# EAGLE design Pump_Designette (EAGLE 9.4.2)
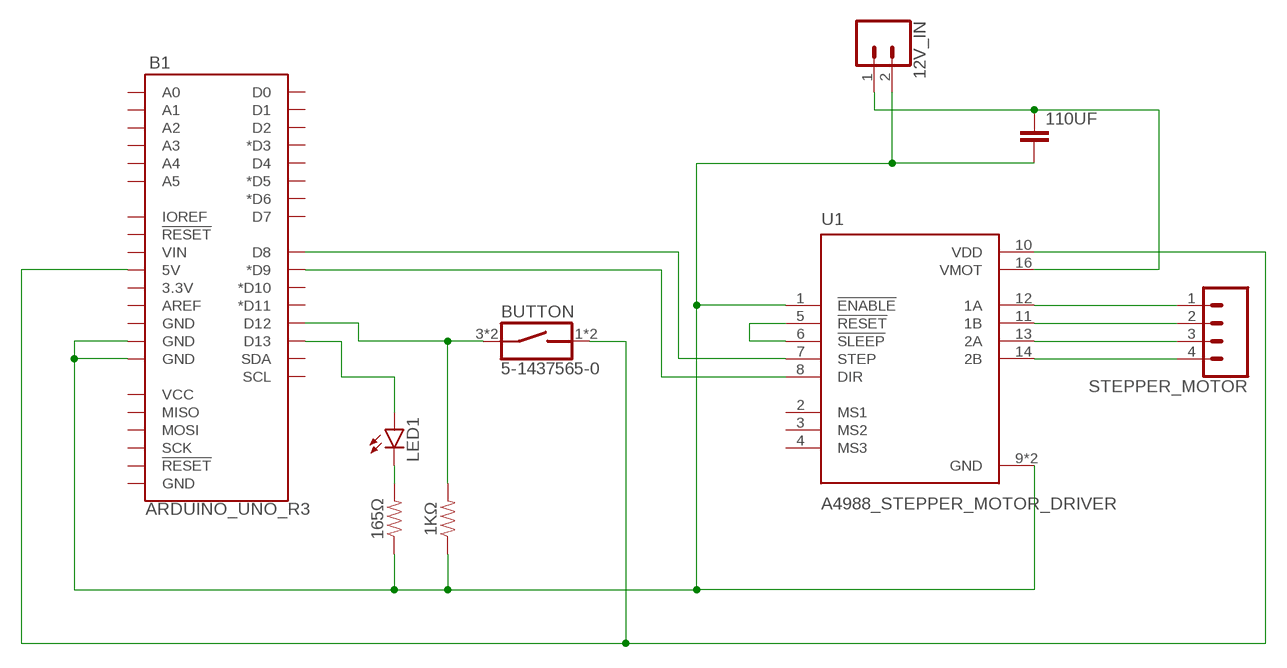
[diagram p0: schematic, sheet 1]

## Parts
1KΩ  1k  1KOHM-HORIZ-1/4W-1%  [AXIAL-0.3]
12V_IN  CONN_02  [1X02]
110UF  C2,5-3  [C2.5-3]
165Ω  1k  1KOHM-HORIZ-1/4W-1%  [AXIAL-0.3]
B1  ARDUINO_UNO_R3  [ARDUINO_R3]
BUTTON  5-1437565-0  [SW_5-1437565-0]
LED1  LED5MM  [LED5MM]
STEPPER_MOTOR  CONN_04  [1X04]
U1  A4988_STEPPER_MOTOR_DRIVER  A4988_STEPPER_MOTOR_DRIVER_CARRIER  [MODULE_A4988_STEPPER_MOTOR_DRIVER_CARRIER]

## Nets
N$1: 1KΩ.P$1 12V_IN.2 110UF.2 165Ω.P$1 B1.GND@2(GND) B1.GND@3(GND) U1.1(!ENABLE) U1.9(GND) U1.15(GND)
N$2: U1.5(!RESET) U1.6(!SLEEP)
N$3: B1.D9(*D9) U1.8(DIR)
N$4: B1.D8 U1.7(STEP)
N$5: STEPPER_MOTOR.1 U1.12(1A)
N$6: STEPPER_MOTOR.2 U1.11(1B)
N$7: STEPPER_MOTOR.3 U1.13(2A)
N$8: STEPPER_MOTOR.4 U1.14(2B)
N$9: 12V_IN.1 110UF.1 U1.16(VMOT)
N$10: B1.5V BUTTON.1 BUTTON.2 U1.10(VDD)
N$11: B1.D13 LED1.A
N$12: 1KΩ.P$2 B1.D12 BUTTON.3 BUTTON.4
N$13: 165Ω.P$2 LED1.K(C)
Unconnected: B1.3.3V B1.A0 B1.A1 B1.A2 B1.A3 B1.A4 B1.A5 B1.AREF B1.D0 B1.D1 B1.D2 B1.D3(*D3) B1.D4 B1.D5(*D5) B1.D6(*D6) B1.D7 B1.D10(*D10) B1.D11(*D11) B1.GND@1(GND) B1.GND@4(GND) B1.IOREF B1.MISO B1.MOSI B1.RESET@1(!RESET!) B1.RESET@2(!RESET!) B1.SCK B1.SCL B1.SDA B1.VCC B1.VIN U1.2(MS1) U1.3(MS2) U1.4(MS3)

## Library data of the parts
1KΩ 165Ω = SparkFun-Resistors:1KOHM: 1kΩ resistor; PROD_ID: RES-12182
12V_IN = SparkFun-Connectors:CONN_02: Multi connection point. Often used as Generic Header-pin footprint for 0.1 inch spaced/style header connections
110UF = capacitor-wima:C: CAPACITOR
B1 = SparkFun-Boards:ARDUINO_UNO_R3: Arduino R3 Footprint with SPI header Arduino Uno R3 Compatible Footprint. Matches PCB size of the original board. SparkFun Products: SAMD21 Dev Breakout RedBoard R3 Stackable Headers
BUTTON = 5-1437565-0:5-1437565-0: Switch Tactile OFF (ON) Round Button Gull Wing 0.05A 12VDC 1.57N SMD T/R; AVAILABILITY: Unavailable; COMMENT: 5-1437565-0; DESCRIPTION: Switch Push Button N.O. SPST Round Button 0.05A 12VDC 1VA Alternate Contact Gull Wing SMD T/R; MF: TE Connectivity; MP: FSM6JSMATR; PACKAGE: None; PRICE: None; TE_PURCHASE_URL: https://www.te.com/usa-en/product-5-1437565-0.html?te_bu=Cor&te_type=disp&te_campaign=seda_glo_cor-seda-global-disp-prtnr-fy19-seda-model-bom-cta_sma-317_1&elqCampaignId=32493
LED1 = led:LED: LED
STEPPER_MOTOR = SparkFun-Connectors:CONN_04: Multi connection point. Often used as Generic Header-pin footprint for 0.1 inch spaced/style header connections On any of the 0.1 inch spaced packages, you can populate with these: Break Away Headers - Straight (PRT-00116) Break Away Male Headers - Right Angle (PRT-00553) Female Headers (PRT-00115)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; PROD_ID: CONN-09696
U1 = A4988_STEPPER_MOTOR_DRIVER_CARRIER:A4988_STEPPER_MOTOR_DRIVER_CARRIER: Stepper motor controler; IC: A4988; 1A; Uin mot: 8÷35V; AVAILABILITY: Unavailable; DESCRIPTION: Stepper Motor Driver; MF: Pololu; MP: A4988 STEPPER MOTOR DRIVER CARRIER; PACKAGE: None; PRICE: None

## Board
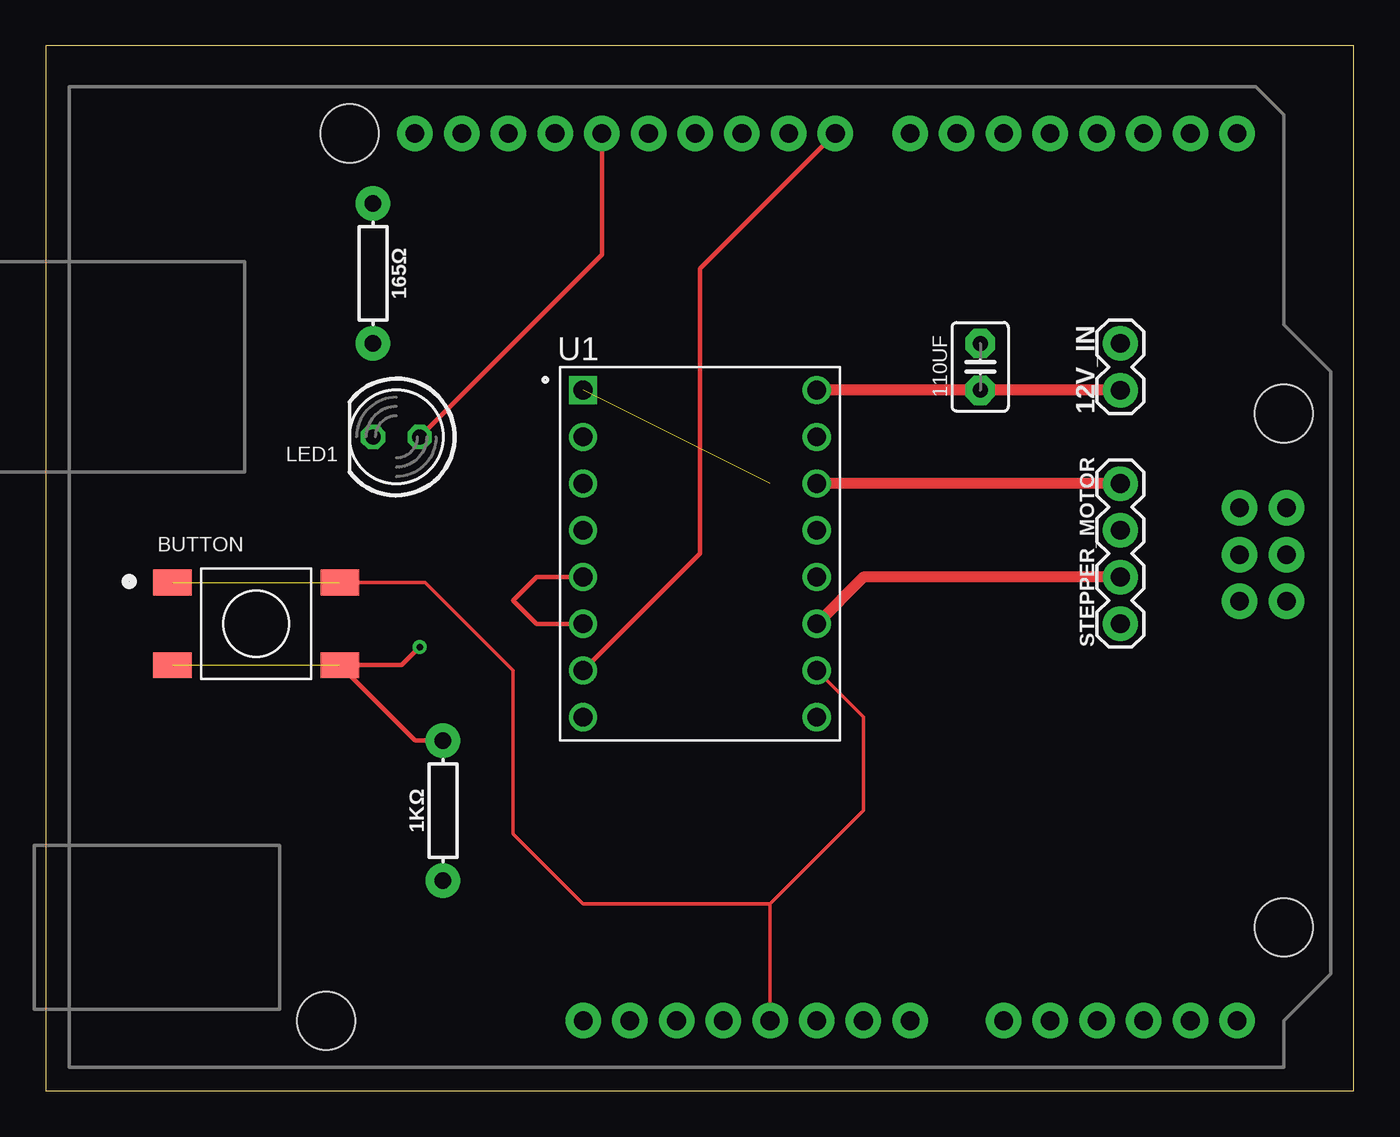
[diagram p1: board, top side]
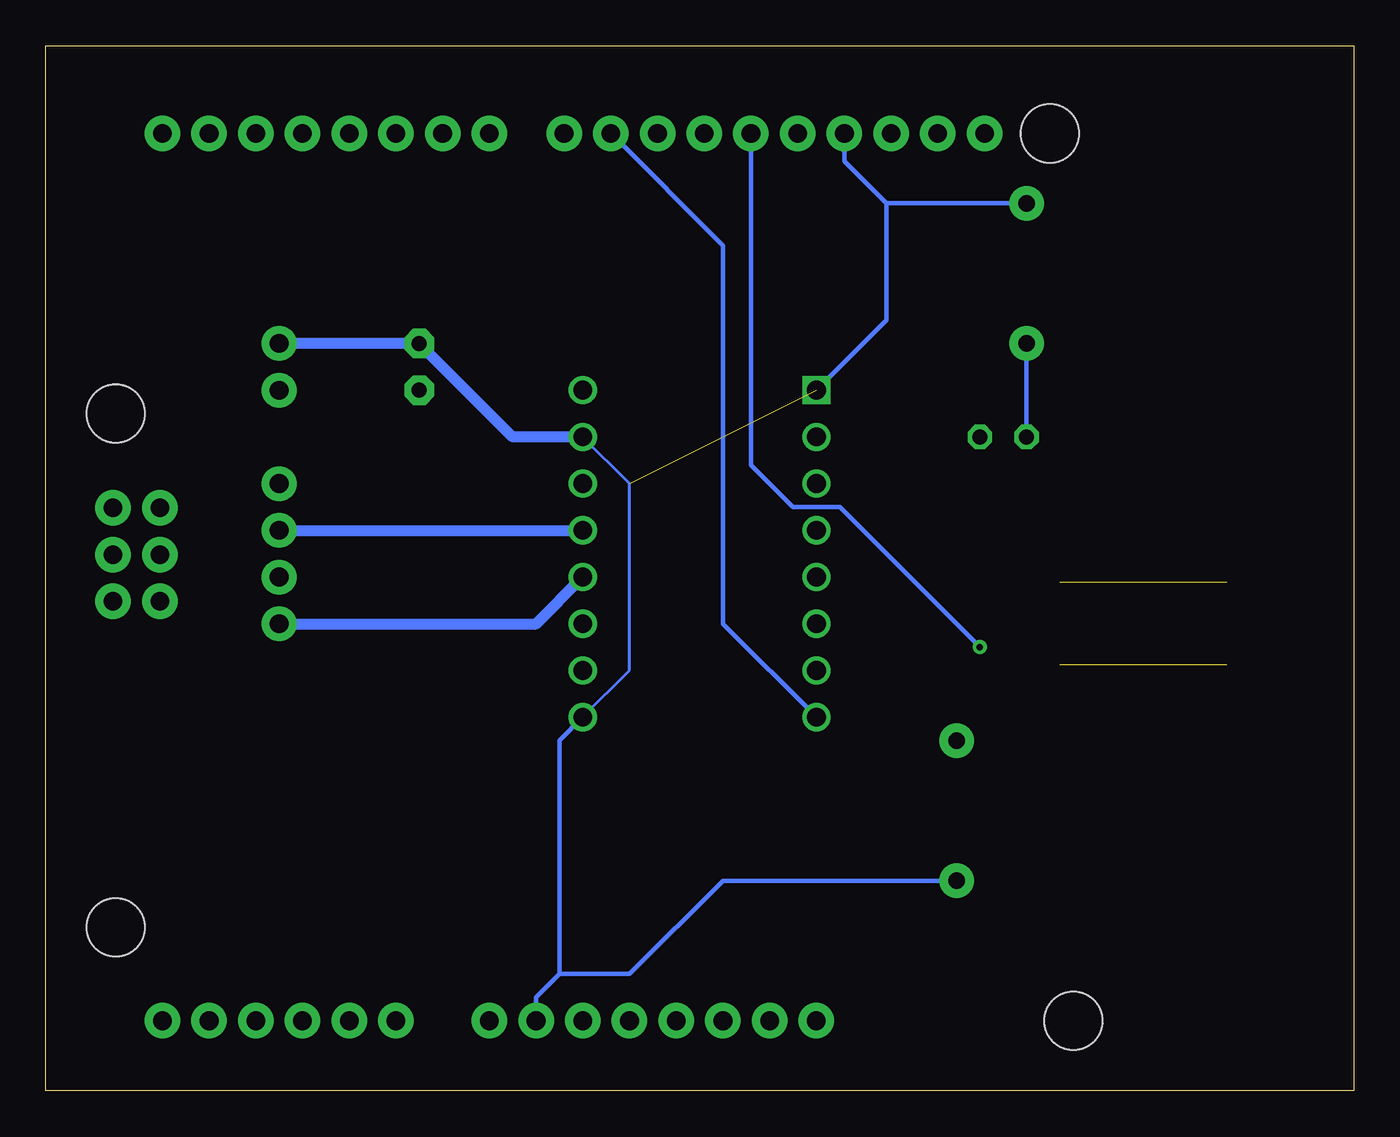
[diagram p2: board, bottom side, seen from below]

Size 71.1 x 56.82 mm. Coordinates in mm from the lower left corner, seen from the top.
Outline: 0,0 71.1,0 71.1,56.82 0,56.82 0,0
Copper layers (1*16): Top 0.035mm / dielectric 1.5mm / Bottom 0.035mm
Design rules "default": minimum track width 6mil, minimum drill 0.35mm, track to track 6mil, track to pad 6mil, pad to pad 6mil, via to via 6mil, smd to smd 6mil, copper to edge 40mil, drill to drill 6mil, minimum pad ring 10mil, minimum via ring 8mil, stop-mask expansion 4mil, vias tented up to drill 0mil, thermal gap 10mil

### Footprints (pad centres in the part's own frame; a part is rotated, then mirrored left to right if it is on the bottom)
AXIAL-0.3 = drill 0.9 pad 1.88: P$1 -3.81,0; P$2 3.81,0
1X02 = drill 1.016 pad 1.88: 1 0,0; 2 2.54,0
C2.5-3 = drill 0.813 pad 1.6 octagon: 1 -1.27,0; 2 1.27,0
ARDUINO_R3 = drill 1.016 pad 1.93: 3.3V 2.54,-24.13; 5V 5.08,-24.13; A0 17.78,-24.13; A1 20.32,-24.13; A2 22.86,-24.13; A3 25.4,-24.13; A4 27.94,-24.13; A5 30.48,-24.13; AREF -9.144,24.13; D0 30.48,24.13; D1 27.94,24.13; D2 25.4,24.13; D3 22.86,24.13; D4 20.32,24.13; D5 17.78,24.13; D6 15.24,24.13; D7 12.7,24.13; D8 8.636,24.13; D9 6.096,24.13; D10 3.556,24.13; D11 1.016,24.13; D12 -1.524,24.13; D13 -4.064,24.13; GND@1 7.62,-24.13; GND@2 10.16,-24.13; GND@3 -6.604,24.13; GND@4 33.16,-1.32; IOREF -2.54,-24.13; MISO 30.62,3.76; MOSI 33.16,1.22; NC -5.08,-24.13; RESET@1 0,-24.13; RESET@2 30.62,-1.32; SCK 30.62,1.22; SCL -14.224,24.13; SDA -11.684,24.13; VCC 33.16,3.76; VIN 12.7,-24.13 | hole 3.175: -17.78,24.13; 33.02,8.89; 33.02,-19.05; -19.05,-24.13
SW_5-1437565-0 = smd 2.1 x 1.4: 1 -4.55,2.25; 2 4.55,2.25; 3 -4.55,-2.25; 4 4.55,-2.25
LED5MM = drill 0.813 octagon: A -1.27,0; K 1.27,0
1X04 = drill 1.016 pad 1.88: 1 0,0; 2 2.54,0; 3 5.08,0; 4 7.62,0
MODULE_A4988_STEPPER_MOTOR_DRIVER_CARRIER = drill 1.02 square: 1 -6.35,8.89 | drill 1.02: 2 -6.35,6.35; 3 -6.35,3.81; 4 -6.35,1.27; 5 -6.35,-1.27; 6 -6.35,-3.81; 7 -6.35,-6.35; 8 -6.35,-8.89; 9 6.35,-8.89; 10 6.35,-6.35; 11 6.35,-3.81; 12 6.35,-1.27; 13 6.35,1.27; 14 6.35,3.81; 15 6.35,6.35; 16 6.35,8.89

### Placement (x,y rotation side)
1KΩ  21.59,15.24 90 top
12V_IN  58.42,38.1 90 top
110UF  50.8,39.37 90 top
165Ω  17.78,44.45 270 top
B1  34.29,27.94 0 top
BUTTON  11.43,25.4 0 top
LED1  19.05,35.56 180 top
STEPPER_MOTOR  58.42,25.4 90 top
U1  35.56,29.21 0 top

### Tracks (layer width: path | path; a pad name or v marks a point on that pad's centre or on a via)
N$1  (1 unrouted)
  Bottom 0.152: U1.9 39.37,22.86 39.37,33.02 U1.15
  Bottom 0.254: 1KΩ.P$1 34.29,11.43 39.37,6.35 43.18,6.35 | 43.18,6.35 44.45,5.08 B1.GND@2 | U1.9 43.18,19.05 43.18,6.35 | B1.GND@3 27.69,50.55 25.4,48.26 | 25.4,48.26 25.4,41.91 U1.1 | 25.4,48.26 165Ω.P$1
  Bottom 0.61: U1.15 45.72,35.56 110UF.2 12V_IN.2
N$2
  Top 0.254: U1.6 26.67,25.4 25.4,26.67 26.67,27.94 U1.5
N$3
  Bottom 0.254: U1.8 34.29,25.4 34.29,45.97 B1.D9
N$4
  Top 0.254: U1.7 35.56,29.21 35.56,44.7 B1.D8
N$5
  Bottom 0.61: STEPPER_MOTOR.1 44.45,25.4 U1.12
N$6
  Top 0.61: STEPPER_MOTOR.2 44.45,27.94 U1.11
N$7
  Bottom 0.61: STEPPER_MOTOR.3 U1.13
N$8
  Top 0.61: STEPPER_MOTOR.4 U1.14
N$9
  Top 0.61: 12V_IN.1 110UF.1 U1.16
N$10  (1 unrouted)
  Top 0.203: B1.5V 39.37,10.16 | 39.37,10.16 44.45,15.24 44.45,20.32 U1.10 | BUTTON.2 20.61,27.65 25.4,22.86 25.4,13.97 29.21,10.16 39.37,10.16
N$11
  Top 0.254: B1.D13 30.23,45.47 LED1.A
N$12  (via drill 0.35)  (1 unrouted)
  Top 0.254: 1KΩ.P$2 20.08,19.05 BUTTON.4 19.34,23.15 v20.32,24.13
  Bottom 0.254: v20.32,24.13 27.94,31.75 30.48,31.75 32.77,34.04 B1.D12
N$13
  Bottom 0.254: 165Ω.P$2 LED1.K

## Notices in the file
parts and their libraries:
SparkFun-Boards: Licensing: Creative Commons ShareAlike 4.0 International - https://creativecommons.org/licenses/by-sa/4.0
